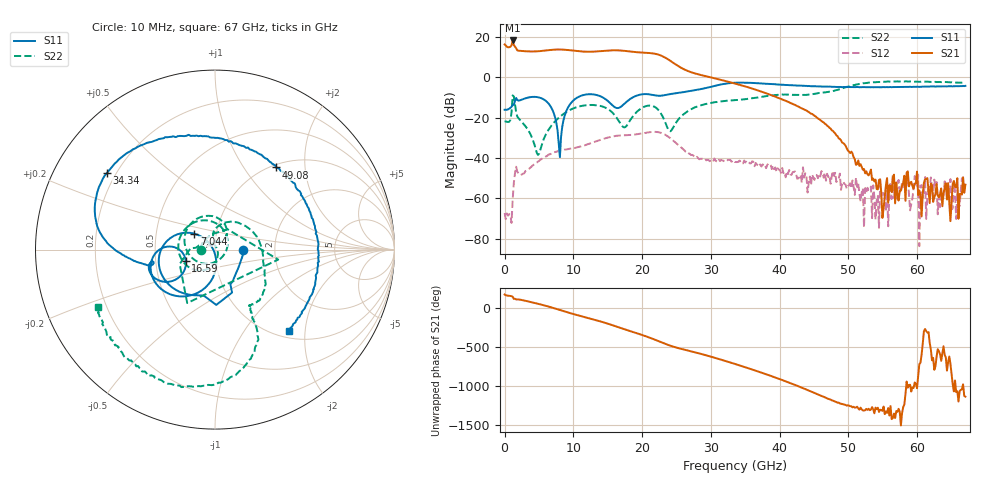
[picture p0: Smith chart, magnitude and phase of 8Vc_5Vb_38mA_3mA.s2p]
! MARKI MICROWAVE INC.
! Date:  05/05/2020
! Model Number:  APM-7099CH
! Description:  2-port Small Signal S-parameter data for APM-7099CH
! Frequency Range:  10 MHz to 67 GHz
! Port Configuration:  PORT 1: Input
!  PORT 2: Output
! Bias Condition: Vc = +8V, Vb = +5V
! APM-7099CH s2p files are only valid for small signal conditions (below -5 dBm input power)
!S2P File: Measurements: Mag<S11> Ang<S11>, Mag<S21> Ang<S21>, Mag<S12> Ang<S12>, Mag<S22> Ang<S22>!row 1
# Hz S  dB  R 50
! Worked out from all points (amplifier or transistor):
!   401 points, 10 MHz to 67 GHz, reference 50 ohm
!   highest |S21| = 18.3 dB at 1.182 GHz (marker M1)
!   |S21| within 3 dB of that: 876.4 MHz to 1.503 GHz (627.1 MHz wide, 52.7 % of centre)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
!   unconditionally stable (mu >= 1): start of sweep to end of sweep
!   at 11.06 GHz: K = 5.06, MAG = 13.6 dB, |S12| = -34.3 dB
!   at 33.51 GHz: K = 38.40, MAG = 0.6 dB, |S12| = -42.0 dB
!   at 67 GHz: K = 29767.20, MAG = -47.9 dB, |S12| = -52.9 dB
!   S11 on the Smith chart (normalised r, x): 10 MHz: 1.37, -0.00; 7.044 GHz: 0.78, +0.14; 16.59 GHz: 0.72, -0.09; 34.34 GHz: 0.17, +0.31; 49.08 GHz: 1.04, +1.41; 67 GHz: 1.13, -1.65
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1e7  -16.09 -0.5  16.29 178.7  -67.26 -2.6  -21.97 -178.6
1.182325e9  -13.82 -61.4  18.27 149.8  -60.68 86.7  -8.96 -9.0
1.68475e9  -10.22 -88.7  14.43 115.5  -44.31 -78.5  -17.27 177.1
4.36435e9  -9.69 -156.5  12.83 70.8  -42.99 -160.9  -33.52 86.4
7.04395e9  -16.77 142.3  13.67 7.4  -37.51 137.0  -22.96 -89.3
9.221125e9  -15.00 -97.6  13.52 -51.8  -35.61 88.1  -16.72 -127.0
1.123082e10  -9.02 -135.6  12.80 -101.7  -34.09 53.1  -14.17 -166.0
1.441285e10  -10.23 179.8  13.11 -179.5  -30.45 -9.7  -14.67 120.3
1.659002e10  -15.18 -159.1  13.35 117.7  -28.91 -63.3  -21.49 32.2
1.80973e10  -11.15 -142.7  12.85 73.4  -28.59 -99.2  -22.23 -102.8
1.993952e10  -8.45 -157.0  12.26 20.1  -27.91 -142.9  -15.24 168.2
2.111185e10  -8.47 -166.8  12.03 -16.4  -27.21 -174.8  -14.01 121.2
2.245165e10  -9.14 -168.3  11.15 -63.2  -27.24 140.5  -16.51 67.9
2.379145e10  -8.50 -166.4  8.86 -109.6  -29.41 95.0  -25.83 57.2
2.513125e10  -7.79 -168.8  5.83 -147.3  -33.19 60.0  -21.55 97.3
2.931812e10  -5.28 -178.9  0.50 116.9  -41.13 19.2  -13.18 34.2
3.3505e10  -2.68 151.7  -3.10 5.8  -41.97 -30.6  -11.28 -9.1
3.434238e10  -2.64 144.8  -3.90 -17.6  -42.16 -42.2  -11.09 -15.0
4.472582e10  -4.40 78.9  -18.18 4.9  -48.24 34.1  -8.37 -58.9
4.908018e10  -4.90 53.5  -32.33 -148.6  -52.57 -70.7  -5.45 -63.7
5.594665e10  -4.86 10.7  -53.57 62.3  -58.12 -33.1  -2.12 -104.4
6.7e10  -4.25 -47.7  -53.23 -54.8  -52.87 -6.3  -2.78 -153.9
